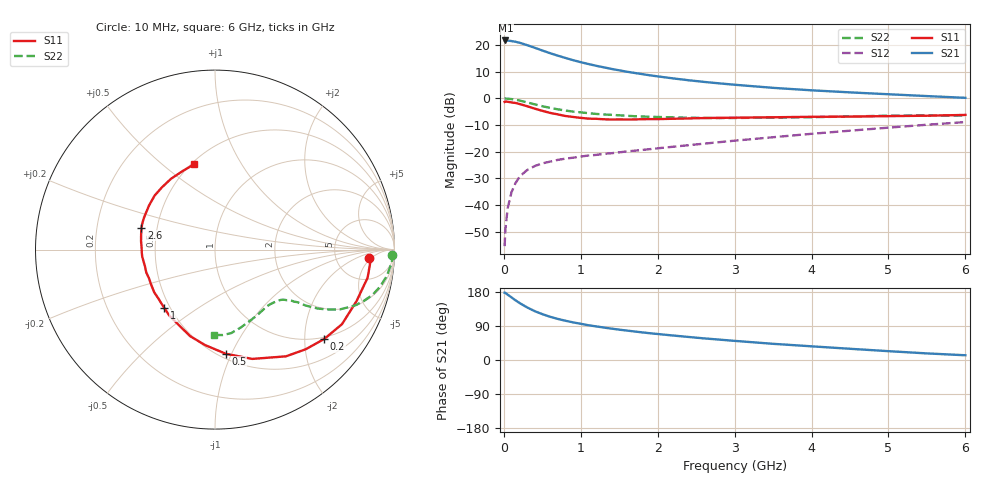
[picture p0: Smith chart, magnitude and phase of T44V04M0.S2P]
! Infineon Technologies  Discrete & RF Semiconductors
! BFR182T
! Si NPN RF Bipolar Junction Transistor in SC75
! VCE = 4 V  IC = 4 mA
! Common Emitter S-Parameters:  October  1999
# GHz  S  MA  R  50
!  f  S11  S21  S12  S22
! GHz  MAG  ANG  MAG  ANG  MAG  ANG  MAG  ANG
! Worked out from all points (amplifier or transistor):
!   36 points, 10 MHz to 6 GHz, reference 50 ohm
!   highest |S21| = 21.7 dB at 20 MHz (marker M1)
!   |S21| within 3 dB of that: start of sweep to 426.8 MHz
!   unconditionally stable (mu >= 1): 1.565 GHz to 4.104 GHz
!   at 250 MHz: K = 0.23, MSG = 24.3 dB, |S12| = -28.2 dB
!   at 1.4 GHz: K = 0.96, MSG = 15.8 dB, |S12| = -20.6 dB
!   at 6 GHz: K = 0.84, MSG = 4.5 dB, |S12| = -8.9 dB
!   S11 on the Smith chart (normalised r, x): 10 MHz: 11, -4; 200 MHz: 0.95, -2.48; 500 MHz: 0.54, -0.95; 1 GHz: 0.46, -0.37; 2.6 GHz: 0.41, +0.12; 6 GHz: 0.52, +0.65
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0.01  0.8568 -3.2  12.14 177.6  0.0017 90.1  0.9845 -1.6
0.02  0.8709 -2.9  12.16 177.1  0.0035 88.7  0.9932 -1.7
0.05  0.8647 -10.4  12.11 172.3  0.0088 87.2  0.9858 -4.5
0.1  0.8392 -20.0  11.84 165.2  0.0175 81.4  0.9688 -8.7
0.15  0.8206 -30.4  11.51 157.7  0.0256 75.0  0.9431 -12.6
0.2  0.7863 -39.3  11.08 151.0  0.0333 71.4  0.9128 -16.1
0.25  0.7508 -47.7  10.51 144.9  0.039 66.6  0.8761 -19.1
0.3  0.714 -56.4  9.961 139.1  0.0451 63.6  0.8422 -21.6
0.4  0.6434 -71.2  8.891 129.0  0.0538 57.9  0.7717 -25.6
0.5  0.5839 -84.0  7.89 121.1  0.0604 54.6  0.7134 -27.9
0.6  0.5352 -95.8  7.031 114.1  0.0652 52.4  0.664 -29.7
0.7  0.5015 -106.1  6.321 108.5  0.0703 51.0  0.6237 -30.8
0.8  0.4672 -115.3  5.722 103.6  0.0742 50.3  0.5921 -31.7
1  0.4311 -131.0  4.762 95.5  0.0812 50.2  0.5465 -32.5
1.1  0.4171 -139.0  4.401 91.7  0.085 50.2  0.5277 -33.3
1.5  0.4035 -161.5  3.349 80.1  0.0974 52.8  0.4816 -35.6
2.2  0.4147 173.5  2.367 64.6  0.124 56.8  0.441 -41.9
2.6  0.4277 163.3  2.036 57.1  0.1415 58.6  0.4299 -46.5
3.5  0.4423 146.1  1.574 42.7  0.187 60.2  0.4353 -57.8
4.5  0.4557 130.5  1.295 29.6  0.2479 58.9  0.4575 -71.9
5.5  0.4732 112.5  1.103 17.4  0.3206 55.0  0.4779 -84.9
6  0.4895 103.8  1.023 12.5  0.3595 51.7  0.4756 -90.6
